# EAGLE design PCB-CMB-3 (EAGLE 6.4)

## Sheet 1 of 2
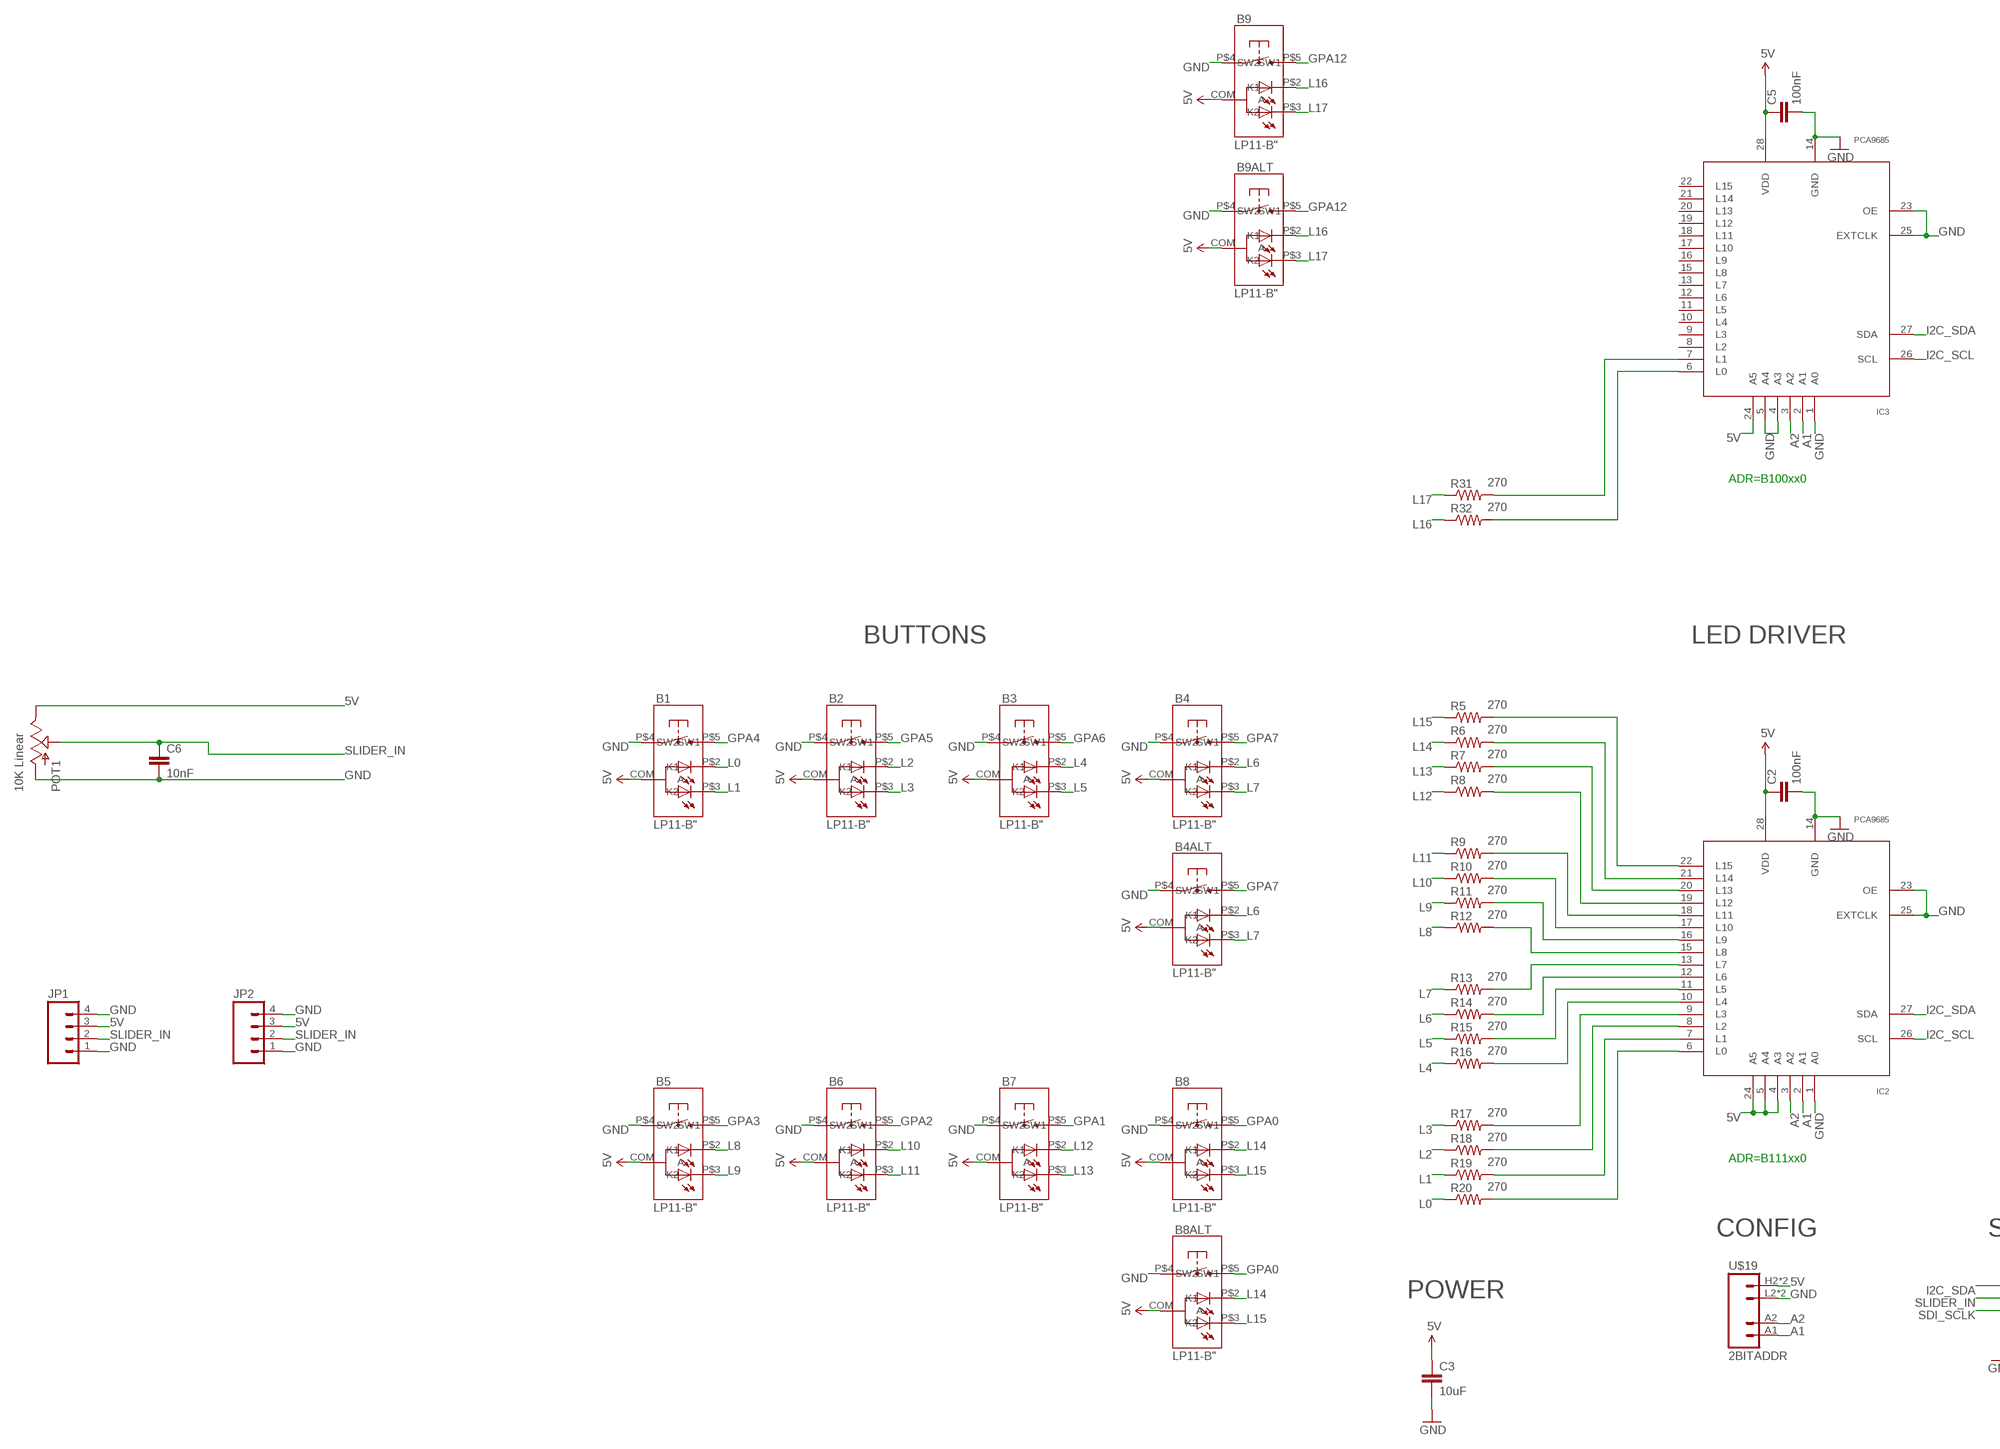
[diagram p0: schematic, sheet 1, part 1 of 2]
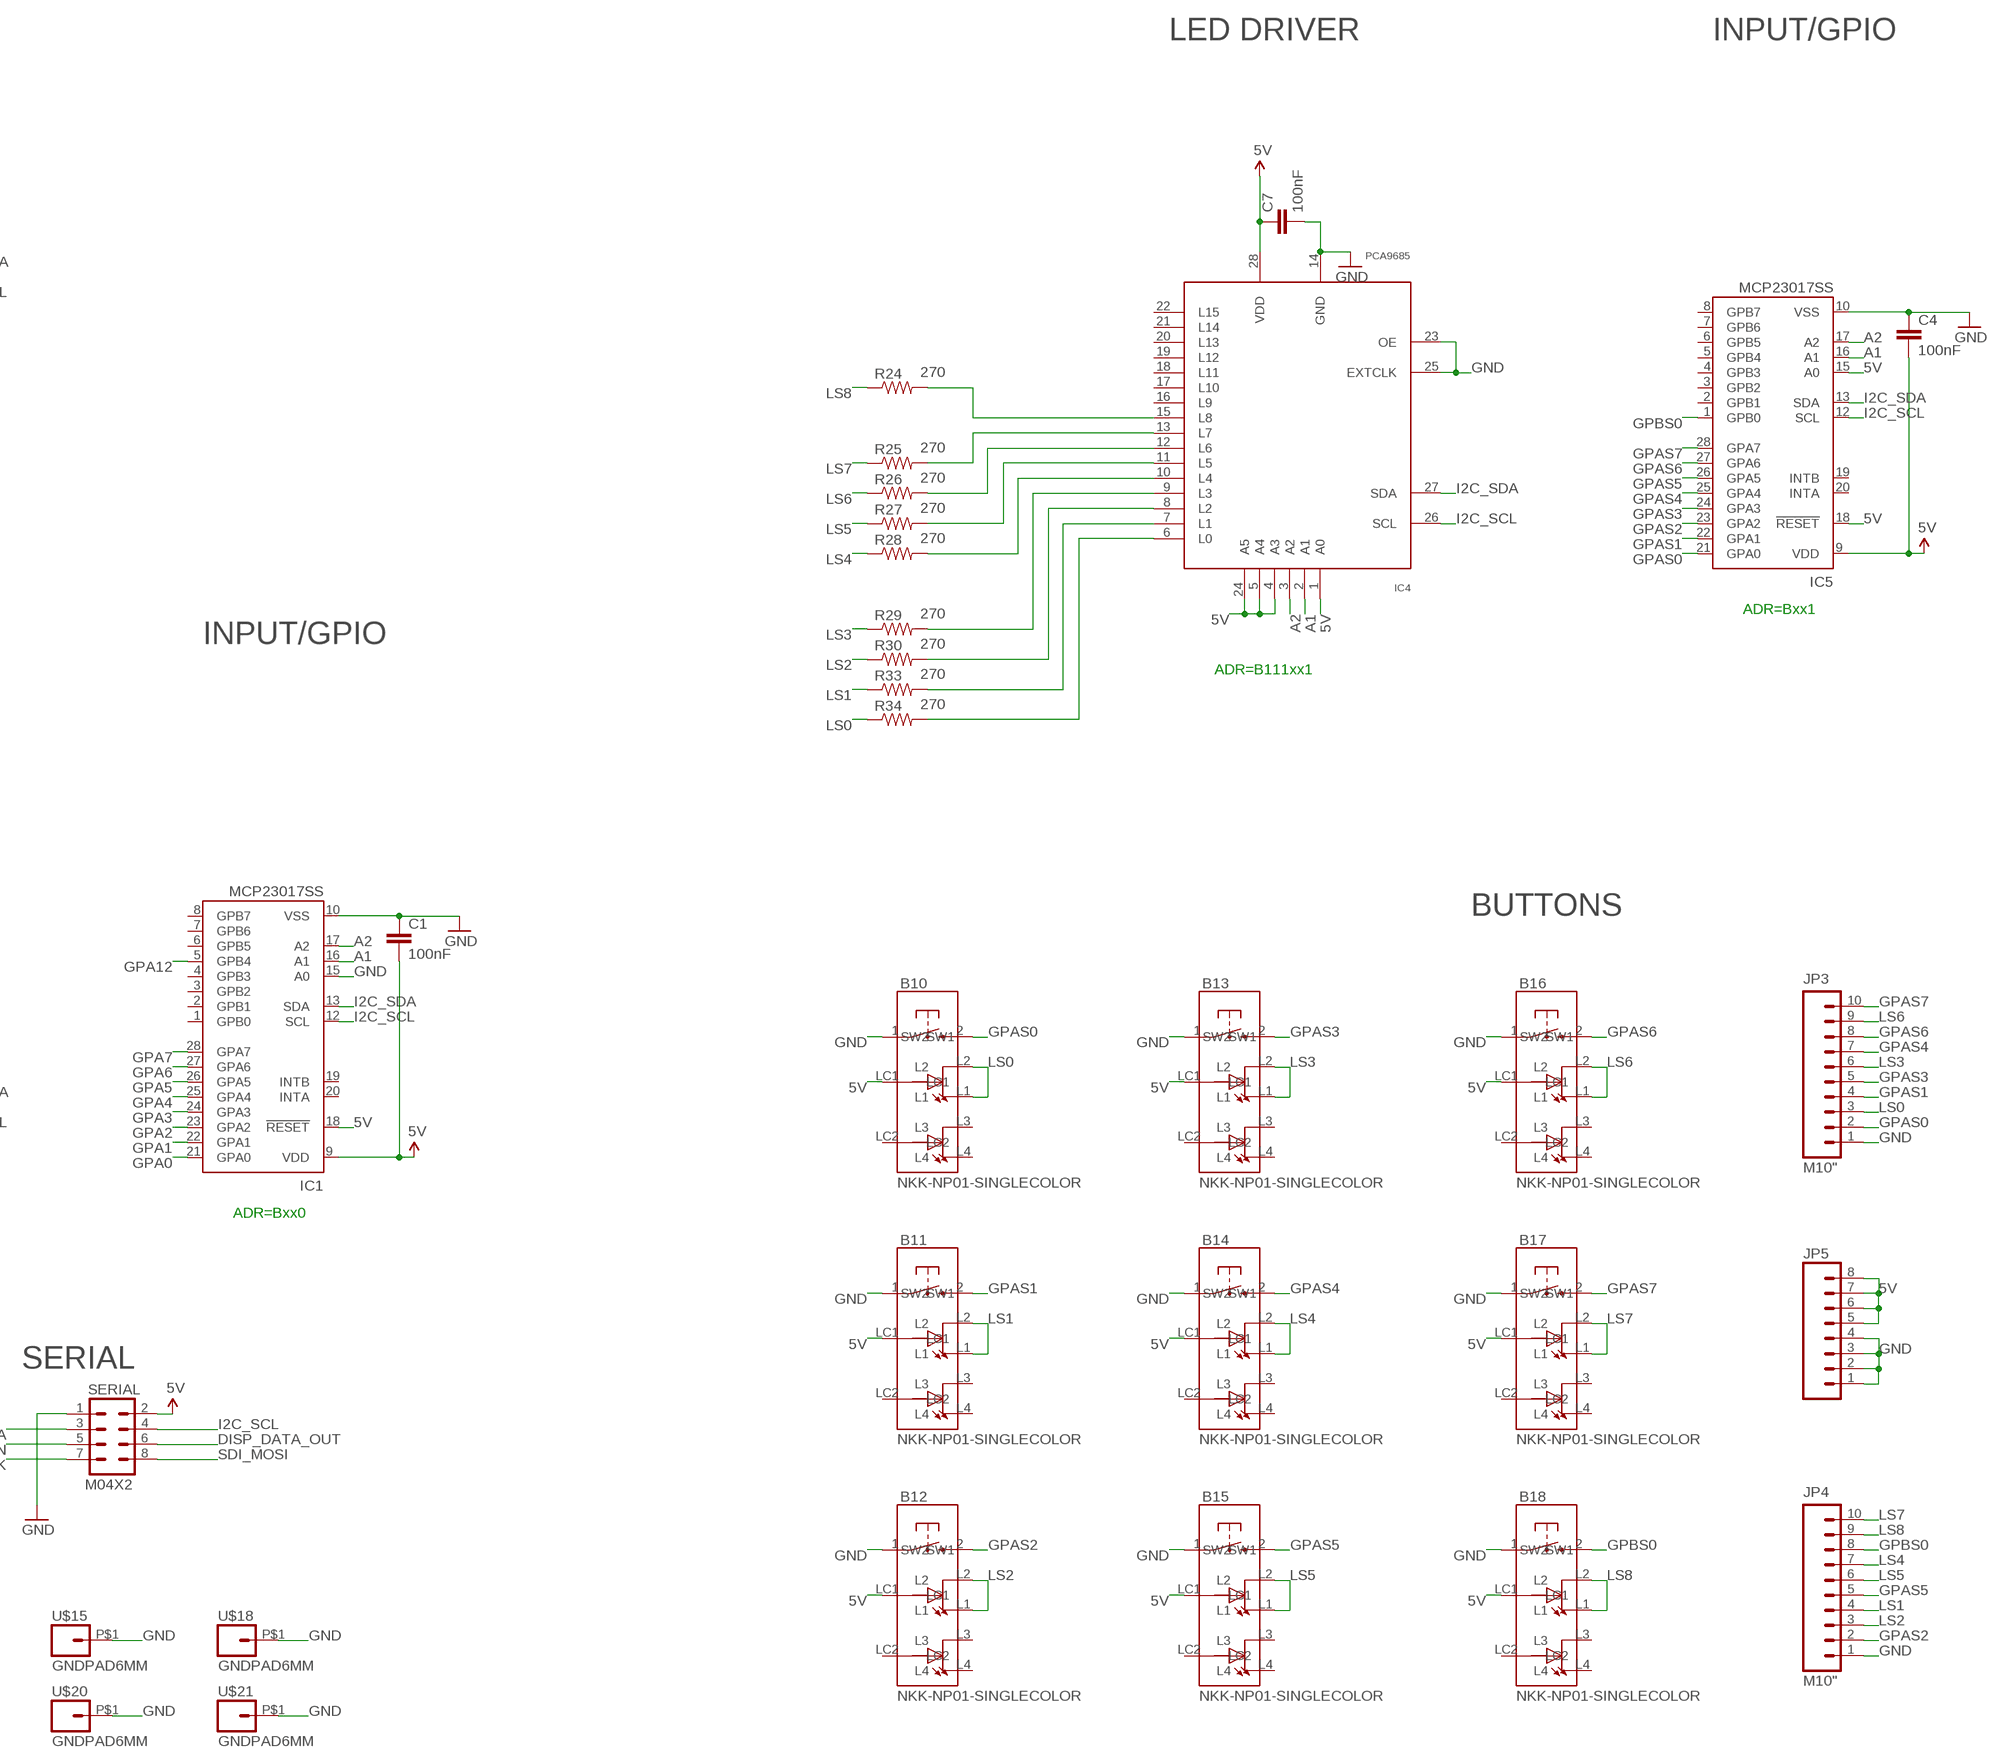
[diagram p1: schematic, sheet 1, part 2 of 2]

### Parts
B1  LP11-B"  [LP11]
B2  LP11-B"  [LP11]
B3  LP11-B"  [LP11]
B4  LP11-B"  [LP11]
B4ALT  LP11-B"  [LP11]
B5  LP11-B"  [LP11]
B6  LP11-B"  [LP11]
B7  LP11-B"  [LP11]
B8  LP11-B"  [LP11]
B8ALT  LP11-B"  [LP11]
B9  LP11-B"  [LP11]
B9ALT  LP11-B"  [LP11]
B10  NKK-NP01-SINGLECOLOR  [NKK-NP01]
B11  NKK-NP01-SINGLECOLOR  [NKK-NP01]
B12  NKK-NP01-SINGLECOLOR  [NKK-NP01]
B13  NKK-NP01-SINGLECOLOR  [NKK-NP01]
B14  NKK-NP01-SINGLECOLOR  [NKK-NP01]
B15  NKK-NP01-SINGLECOLOR  [NKK-NP01]
B16  NKK-NP01-SINGLECOLOR  [NKK-NP01]
B17  NKK-NP01-SINGLECOLOR  [NKK-NP01]
B18  NKK-NP01-SINGLECOLOR  [NKK-NP01]
C1  100nF  CAP0603-CAP  [0603-CAP]
C2  100nF  CAP0603-CAP  [0603-CAP]
C3  10uF  CAP0805  [0805]
C4  100nF  CAP0603-CAP  [0603-CAP]
C5  100nF  CAP0603-CAP  [0603-CAP]
C6  10nF  CAP0603-CAP  [0603-CAP]
C7  100nF  CAP0603-CAP  [0603-CAP]
IC1  MCP23017SS  [SSOP28]
IC2  PCA9685  [TSSOP28]
IC3  PCA9685  [TSSOP28]
IC4  PCA9685  [TSSOP28]
IC5  MCP23017SS  [SSOP28]
JP1  M04PTH  [1X04]
JP2  M04PTH  [1X04]
JP3  M10"  [1X10]
JP4  M10"  [1X10]
JP5  M08LOCK  [1X08_LOCK]
POT1  10K Linear  SLIDER20  [SLIDER20]
R5  270  RESISTOR0603-RES  [0603-RES]
R6  270  RESISTOR0603-RES  [0603-RES]
R7  270  RESISTOR0603-RES  [0603-RES]
R8  270  RESISTOR0603-RES  [0603-RES]
R9  270  RESISTOR0603-RES  [0603-RES]
R10  270  RESISTOR0603-RES  [0603-RES]
R11  270  RESISTOR0603-RES  [0603-RES]
R12  270  RESISTOR0603-RES  [0603-RES]
R13  270  RESISTOR0603-RES  [0603-RES]
R14  270  RESISTOR0603-RES  [0603-RES]
R15  270  RESISTOR0603-RES  [0603-RES]
R16  270  RESISTOR0603-RES  [0603-RES]
R17  270  RESISTOR0603-RES  [0603-RES]
R18  270  RESISTOR0603-RES  [0603-RES]
R19  270  RESISTOR0603-RES  [0603-RES]
R20  270  RESISTOR0603-RES  [0603-RES]
R24  270  RESISTOR0603-RES  [0603-RES]
R25  270  RESISTOR0603-RES  [0603-RES]
R26  270  RESISTOR0603-RES  [0603-RES]
R27  270  RESISTOR0603-RES  [0603-RES]
R28  270  RESISTOR0603-RES  [0603-RES]
R29  270  RESISTOR0603-RES  [0603-RES]
R30  270  RESISTOR0603-RES  [0603-RES]
R31  270  RESISTOR0603-RES  [0603-RES]
R32  270  RESISTOR0603-RES  [0603-RES]
R33  270  RESISTOR0603-RES  [0603-RES]
R34  270  RESISTOR0603-RES  [0603-RES]
SERIAL  M04X2  [2X4]
U$15  GNDPAD6MM  [3.2MMPAD6MM]
U$18  GNDPAD6MM  [3.2MMPAD6MM]
U$19  2BITADDR  [2BITADDR]
U$20  GNDPAD6MM  [3.2MMPAD6MM]
U$21  GNDPAD6MM  [3.2MMPAD6MM]

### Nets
5V [Power]: B1.COM(A) B2.COM(A) B3.COM(A) B4.COM(A) B4ALT.COM(A) B5.COM(A) B6.COM(A) B7.COM(A) B8.COM(A) B8ALT.COM(A) B9.COM(A) B9ALT.COM(A) B10.LC1 B11.LC1 B12.LC1 B13.LC1 B14.LC1 B15.LC1 B16.LC1 B17.LC1 B18.LC1 C1.2 C2.1 C3.1 C4.2 C5.1 C7.1 IC1.9(VDD) IC1.18(!RESET) IC2.4(A3) IC2.5(A4) IC2.24(A5) IC2.28(VDD) IC3.24(A5) IC3.28(VDD) IC4.1(A0) IC4.4(A3) IC4.5(A4) IC4.24(A5) IC4.28(VDD) IC5.9(VDD) IC5.15(A0) IC5.18(!RESET) JP1.3 JP2.3 JP5.5 JP5.6 JP5.7 JP5.8 POT1.1(E) SERIAL.2 U$19.H2(VCC) U$19.H3(VCC)
A1: IC1.16(A1) IC2.2(A1) IC3.2(A1) IC4.2(A1) IC5.16(A1) U$19.A1
A2: IC1.17(A2) IC2.3(A2) IC3.3(A2) IC4.3(A2) IC5.17(A2) U$19.A2
DISP_DATA_OUT: SERIAL.6
GND [Power]: B1.P$4(SW1) B2.P$4(SW1) B3.P$4(SW1) B4.P$4(SW1) B4ALT.P$4(SW1) B5.P$4(SW1) B6.P$4(SW1) B7.P$4(SW1) B8.P$4(SW1) B8ALT.P$4(SW1) B9.P$4(SW1) B9ALT.P$4(SW1) B10.1(SW1) B11.1(SW1) B12.1(SW1) B13.1(SW1) B14.1(SW1) B15.1(SW1) B16.1(SW1) B17.1(SW1) B18.1(SW1) C1.1 C2.2 C3.2 C4.1 C5.2 C6.2 C7.2 IC1.10(VSS) IC1.15(A0) IC2.1(A0) IC2.14(GND) IC2.23(OE) IC2.25(EXTCLK) IC3.1(A0) IC3.4(A3) IC3.5(A4) IC3.14(GND) IC3.23(OE) IC3.25(EXTCLK) IC4.14(GND) IC4.23(OE) IC4.25(EXTCLK) IC5.10(VSS) JP1.1 JP1.4 JP2.1 JP2.4 JP3.1 JP4.1 JP5.1 JP5.2 JP5.3 JP5.4 POT1.3(A) SERIAL.1 U$15.P$1 U$18.P$1 U$19.L2(GND) U$19.L3(GND) U$20.P$1 U$21.P$1
GPA0: B8.P$5(SW2) B8ALT.P$5(SW2) IC1.21(GPA0)
GPA1: B7.P$5(SW2) IC1.22(GPA1)
GPA2: B6.P$5(SW2) IC1.23(GPA2)
GPA3: B5.P$5(SW2) IC1.24(GPA3)
GPA4: B1.P$5(SW2) IC1.25(GPA4)
GPA5: B2.P$5(SW2) IC1.26(GPA5)
GPA6: B3.P$5(SW2) IC1.27(GPA6)
GPA7: B4.P$5(SW2) B4ALT.P$5(SW2) IC1.28(GPA7)
GPA12: B9.P$5(SW2) B9ALT.P$5(SW2) IC1.5(GPB4)
GPAS0: B10.2(SW2) IC5.21(GPA0) JP3.2
GPAS1: B11.2(SW2) IC5.22(GPA1) JP3.4
GPAS2: B12.2(SW2) IC5.23(GPA2) JP4.2
GPAS3: B13.2(SW2) IC5.24(GPA3) JP3.5
GPAS4: B14.2(SW2) IC5.25(GPA4) JP3.7
GPAS5: B15.2(SW2) IC5.26(GPA5) JP4.5
GPAS6: B16.2(SW2) IC5.27(GPA6) JP3.8
GPAS7: B17.2(SW2) IC5.28(GPA7) JP3.10
GPBS0 [Power]: B18.2(SW2) IC5.1(GPB0) JP4.8
I2C_SCL: IC1.12(SCL) IC2.26(SCL) IC3.26(SCL) IC4.26(SCL) IC5.12(SCL) SERIAL.4
I2C_SDA: IC1.13(SDA) IC2.27(SDA) IC3.27(SDA) IC4.27(SDA) IC5.13(SDA) SERIAL.3
L0: B1.P$2(K1) R20.1
L1: B1.P$3(K2) R19.1
L2: B2.P$2(K1) R18.1
L3: B2.P$3(K2) R17.1
L4: B3.P$2(K1) R16.1
L5: B3.P$3(K2) R15.1
L6: B4.P$2(K1) B4ALT.P$2(K1) R14.1
L7: B4.P$3(K2) B4ALT.P$3(K2) R13.1
L8: B5.P$2(K1) R12.1
L9: B5.P$3(K2) R11.1
L10: B6.P$2(K1) R10.1
L11: B6.P$3(K2) R9.1
L12: B7.P$2(K1) R8.1
L13: B7.P$3(K2) R7.1
L14: B8.P$2(K1) B8ALT.P$2(K1) R6.1
L15: B8.P$3(K2) B8ALT.P$3(K2) R5.1
L16: B9.P$2(K1) B9ALT.P$2(K1) R32.1
L17: B9.P$3(K2) B9ALT.P$3(K2) R31.1
LS0: B10.L1 B10.L2 JP3.3 R34.1
LS1: B11.L1 B11.L2 JP4.4 R33.1
LS2: B12.L1 B12.L2 JP4.3 R30.1
LS3: B13.L1 B13.L2 JP3.6 R29.1
LS4: B14.L1 B14.L2 JP4.7 R28.1
LS5: B15.L1 B15.L2 JP4.6 R27.1
LS6: B16.L1 B16.L2 JP3.9 R26.1
LS7: B17.L1 B17.L2 JP4.10 R25.1
LS8: B18.L1 B18.L2 JP4.9 R24.1
N$1: IC4.13(L7) R25.2
N$2: IC4.12(L6) R26.2
N$3: IC4.11(L5) R27.2
N$4: IC2.13(L7) R13.2
N$5: IC2.12(L6) R14.2
N$6: IC4.10(L4) R28.2
N$7: IC2.11(L5) R15.2
N$8: IC4.9(L3) R29.2
N$9: IC2.10(L4) R16.2
N$10: IC2.9(L3) R17.2
N$11: IC2.8(L2) R18.2
N$12: IC2.7(L1) R19.2
N$13: IC4.8(L2) R30.2
N$14: IC3.7(L1) R31.2
N$15: IC3.6(L0) R32.2
N$16: IC4.7(L1) R33.2
N$17: IC4.6(L0) R34.2
N$18: IC4.15(L8) R24.2
N$19: IC2.6(L0) R20.2
N$20: IC2.15(L8) R12.2
N$21: IC2.16(L9) R11.2
N$22: IC2.17(L10) R10.2
N$23: IC2.18(L11) R9.2
N$24: IC2.19(L12) R8.2
N$25: IC2.20(L13) R7.2
N$26: IC2.21(L14) R6.2
N$27: IC2.22(L15) R5.2
SDI_MOSI: SERIAL.8
SDI_SCLK: SERIAL.7
SLIDER_IN: C6.1 JP1.2 JP2.2 POT1.2A(S) SERIAL.5
Unconnected: B10.L3 B10.L4 B10.LC2 B11.L3 B11.L4 B11.LC2 B12.L3 B12.L4 B12.LC2 B13.L3 B13.L4 B13.LC2 B14.L3 B14.L4 B14.LC2 B15.L3 B15.L4 B15.LC2 B16.L3 B16.L4 B16.LC2 B17.L3 B17.L4 B17.LC2 B18.L3 B18.L4 B18.LC2 IC1.1(GPB0) IC1.2(GPB1) IC1.3(GPB2) IC1.4(GPB3) IC1.6(GPB5) IC1.7(GPB6) IC1.8(GPB7) IC1.19(INTB) IC1.20(INTA) IC3.8(L2) IC3.9(L3) IC3.10(L4) IC3.11(L5) IC3.12(L6) IC3.13(L7) IC3.15(L8) IC3.16(L9) IC3.17(L10) IC3.18(L11) IC3.19(L12) IC3.20(L13) IC3.21(L14) IC3.22(L15) IC4.16(L9) IC4.17(L10) IC4.18(L11) IC4.19(L12) IC4.20(L13) IC4.21(L14) IC4.22(L15) IC5.2(GPB1) IC5.3(GPB2) IC5.4(GPB3) IC5.5(GPB4) IC5.6(GPB5) IC5.7(GPB6) IC5.8(GPB7) IC5.19(INTB) IC5.20(INTA)

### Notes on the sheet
- LED DRIVER | INPUT/GPIO
- ADR=B100xx0
- ADR=Bxx1
- BUTTONS | LED DRIVER | INPUT/GPIO
- ADR=B111xx1
- BUTTONS
- ADR=Bxx0
- ADR=B111xx0
- CONFIG | SERIAL
- POWER

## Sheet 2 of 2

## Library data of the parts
B1-B4 B4ALT B5-B8 B8ALT B9 B9ALT = SKAARHOJ:LP11-B
B10-B18 = SKAARHOJ:NKK-NP01-SINGLECOLOR
C1-C7 = SparkFun:CAP: Capacitor
IC1 IC5 = microchip:MCP23017: http://ww1.microchip.com/downloads/en/DeviceDoc/21952a.pdf Source: http://ww1.microchip.com/downloads/en/DeviceDoc/21952a.pdf; MF: MICROCHIP; MPN: MCP23017-E/SS; OC_FARNELL: 1467674; OC_NEWARK: 31K2960
IC2-IC4 = wsmith:PCA9685
JP1 JP2 = SparkFun:M04: Header 4 Standard 4-pin 0.1" header. Use with straight break away headers (SKU : PRT-00116), right angle break away headers (PRT-00553), swiss pins (PRT-00743), machine pins (PRT-00117), and female headers (PRT-00115). Molex polarized connector foot print use with SKU : PRT-08231 with associated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
JP3 JP4 = SparkFun:M10: Header 10 Standard 10-pin 0.1" header. Use with straight break away headers (SKU : PRT-00116), right angle break away headers (PRT-00553), swiss pins (PRT-00743), machine pins (PRT-00117), and female headers (PRT-00115).
JP5 = SparkFun:M08: Header 8 Standard 8-pin 0.1" header. Use with straight break away headers (SKU : PRT-00116), right angle break away headers (PRT-00553), swiss pins (PRT-00743), machine pins (PRT-00117), and female headers (PRT-00115).
POT1 = SKAARHOJ:SLIDER
R5-R20 R24-R34 = SparkFun:RESISTOR: Resistor
SERIAL = SparkFun:M04X2
U$15 U$18 U$20 U$21 = SKAARHOJ:GNDPAD
U$19 = SKAARHOJ:2BITADDR

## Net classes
0 default: width 0.203 mm, drill 0.406 mm, clearance 0.203 mm
1 Power: width 0.406 mm, drill 0.61 mm, clearance 0.203 mm

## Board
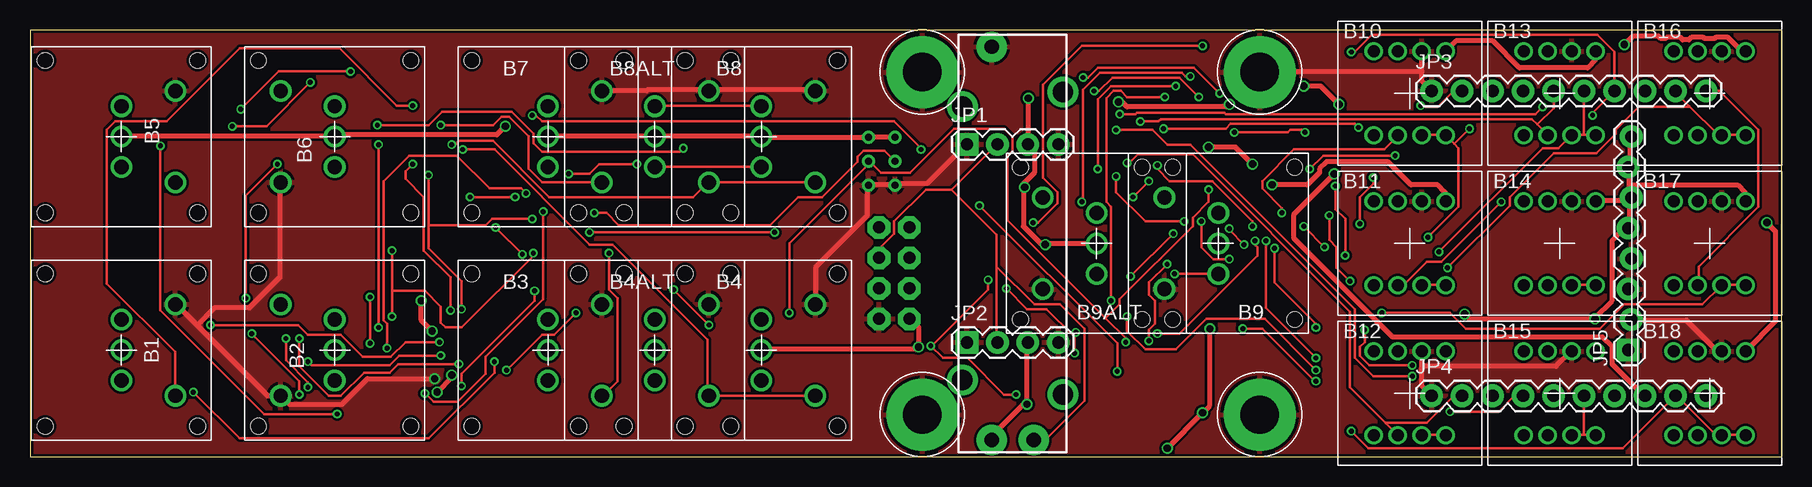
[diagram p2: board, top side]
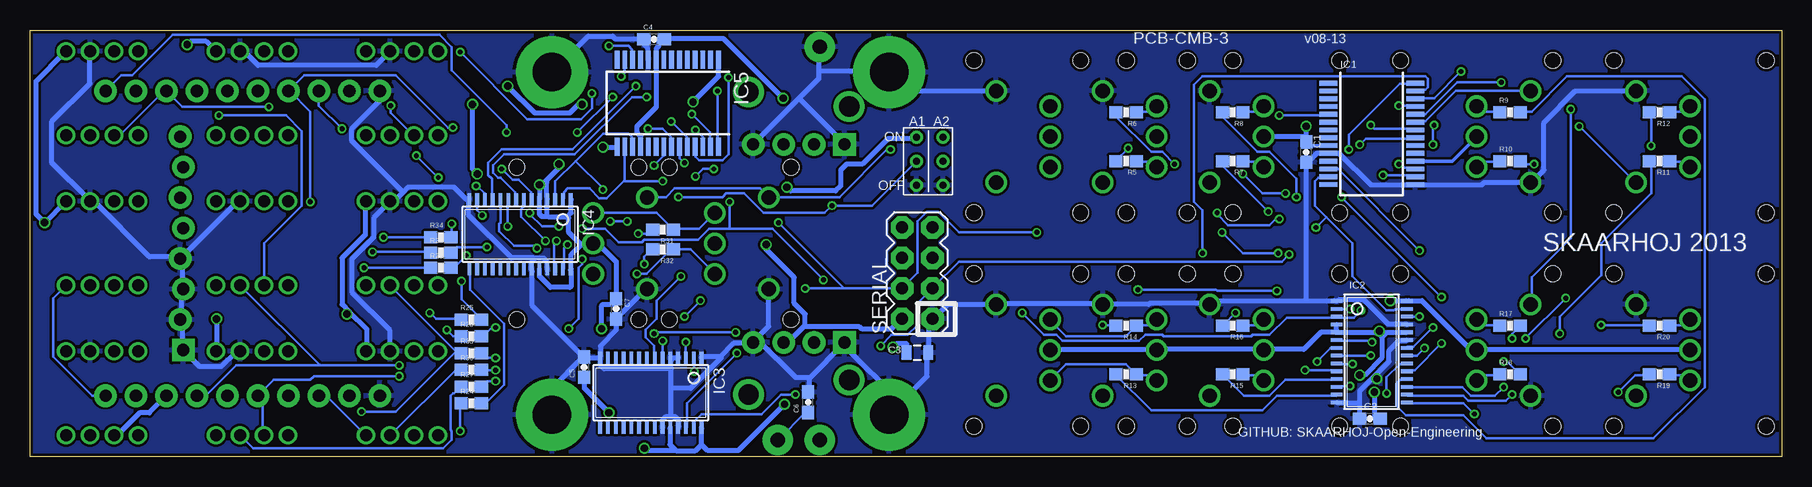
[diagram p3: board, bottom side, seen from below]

Size 146 x 35.56 mm. Coordinates in mm from the lower left corner, seen from the top.
Outline: 0,0 146,0 146,35.56 0,35.56 0,0
Copper layers (1*16): Top 0.035mm / dielectric 1.5mm / Bottom 0.035mm
Design rules "Fusion_eagle_rule_v1.1": minimum track width 6mil, minimum drill 12mil, track to track 6mil, track to pad 6mil, pad to pad 6mil, via to via 6mil, smd to smd 0mil, copper to edge 10mil, drill to drill 10mil, minimum pad ring 10mil, minimum via ring 6mil, stop-mask expansion 2mil, vias tented up to drill 100mil, thermal gap 10mil

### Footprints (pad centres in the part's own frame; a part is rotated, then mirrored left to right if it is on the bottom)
LP11 = drill 1.2: COM 0,0; P$2 0,2.54; P$3 0,-2.54; P$4 4.5,3.81; P$5 4.5,-3.81 | hole 1.3: -6.35,6.35; 6.35,6.35; 6.35,-6.35; -6.35,-6.35
NKK-NP01 = drill 1: 1 1,3.5; 2 -1,-3.5; L1 3,-3.5; L2 1,-3.5; L3 -1,3.5; L4 -3,3.5; LC1 3,3.5; LC2 -3,-3.5
0603-CAP = smd 1.1 x 1: 1 -0.85,0; 2 0.85,0
0805 = smd 0.8 x 1.2: 1 -0.9,0; 2 0.9,0
SSOP28 = smd 0.4 x 1.5: 1 -4.225,-3.625; 2 -3.575,-3.625; 3 -2.925,-3.625; 4 -2.275,-3.625; 5 -1.625,-3.625; 6 -0.975,-3.625; 7 -0.325,-3.625; 8 0.325,-3.625; 9 0.975,-3.625; 10 1.625,-3.625; 11 2.275,-3.625; 12 2.925,-3.625; 13 3.575,-3.625; 14 4.225,-3.625; 15 4.225,3.625; 16 3.575,3.625; 17 2.925,3.625; 18 2.275,3.625; 19 1.625,3.625; 20 0.975,3.625; 21 0.325,3.625; 22 -0.325,3.625; 23 -0.975,3.625; 24 -1.625,3.625; 25 -2.275,3.625; 26 -2.925,3.625; 27 -3.575,3.625; 28 -4.225,3.625
TSSOP28 = smd 0.305 x 0.991: 1 -4.225,-2.918; 2 -3.575,-2.918; 3 -2.925,-2.918; 4 -2.275,-2.918; 5 -1.625,-2.918; 6 -0.975,-2.918; 7 -0.325,-2.918; 8 0.325,-2.918; 9 0.975,-2.918; 10 1.625,-2.918; 11 2.275,-2.918; 12 2.925,-2.918; 13 3.575,-2.918; 14 4.225,-2.918; 15 4.225,2.918; 16 3.575,2.918; 17 2.925,2.918; 18 2.275,2.918; 19 1.625,2.918; 20 0.975,2.918; 21 0.325,2.918; 22 -0.325,2.918; 23 -0.975,2.918; 24 -1.625,2.918; 25 -2.275,2.918; 26 -2.925,2.918; 27 -3.575,2.918; 28 -4.225,2.918
1X04 = drill 1.016 pad 1.88 square: 1 0,0 | drill 1.016 pad 1.88: 2 2.54,0; 3 5.08,0; 4 7.62,0
1X10 = drill 1.016 pad 1.88: 1 0,0; 2 2.54,0; 3 5.08,0; 4 7.62,0; 5 10.16,0; 6 12.7,0; 7 15.24,0; 8 17.78,0; 9 20.32,0; 10 22.86,0
1X08_LOCK = drill 1.016 pad 1.88 square: 1 0,0.127 | drill 1.016 pad 1.88: 2 2.54,-0.127; 3 5.08,0.127; 4 7.62,-0.127; 5 10.16,0.127; 6 12.7,-0.127; 7 15.24,0.127; 8 17.78,-0.127
SLIDER20 = drill 1.194 pad 2.54: 1 -16.383,1.74; 2A -16.383,-1.74; 3 16.383,1.74 | drill 1.702: P$1 -11.392,4.191; P$2 11.392,4.191; P$3 12.598,-4.191; P$4 -12.598,-4.191
0603-RES = smd 1.1 x 1: 1 -0.85,0; 2 0.85,0
2X4 = drill 1.016 pad 1.88 octagon: 1 -3.81,-1.27; 2 -3.81,1.27; 3 -1.27,-1.27; 4 -1.27,1.27; 5 1.27,-1.27; 6 1.27,1.27; 7 3.81,-1.27; 8 3.81,1.27
3.2MMPAD6MM = drill 3.2 pad 6: P$1 0,0
2BITADDR = drill 0.6: A1 0,0; A2 2.2,0; H2 0,2; H3 2.2,2; L2 0,-2; L3 2.2,-2

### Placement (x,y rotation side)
B1  7.62,8.89 0 top
B2  25.4,8.89 180 top
B3  43.18,8.89 0 top
B4  60.96,8.89 0 top
B4ALT  52.07,8.89 0 top
B5  7.62,26.67 0 top
B6  25.4,26.67 180 top
B7  43.18,26.67 0 top
B8  60.96,26.67 0 top
B8ALT  52.07,26.67 0 top
B9  99.06,17.78 180 top
B9ALT  88.9,17.78 180 top
B10  115,30.28 0 top
B11  115,17.78 0 top
B12  115,5.28 0 top
B13  127.5,30.28 0 top
B14  127.5,17.78 0 top
B15  127.5,5.28 0 top
B16  140,30.28 0 top
B17  140,17.78 0 top
B18  140,5.28 0 top
C1  39.62,25.38 90 bottom
C2  34.32,3.16 180 bottom
C3  72.04,8.67 0 bottom
C4  93.98,34.8 0 bottom
C5  99.81,7.47 90 bottom
C6  81.13,4.54 90 bottom
C7  97.16,12.32 270 bottom
IC1  34.16,26.91 270 bottom
IC2  34.16,8.75 270 bottom
IC3  94.25,5.33 180 bottom
IC4  105.16,18.54 180 bottom
IC5  92.84,29.46 180 bottom
JP1  78.11,26.04 0 top
JP2  78.11,9.53 0 top
JP3  116.84,30.48 0 top
JP4  116.84,5.08 0 top
JP5  133.35,8.89 90 top
POT1  81.92,17.78 90 top
R5  54.63,24.64 180 bottom
R6  54.63,28.7 180 bottom
R7  45.74,24.64 180 bottom
R8  45.74,28.7 180 bottom
R9  22.62,28.7 0 bottom
R10  22.62,24.64 0 bottom
R11  10.18,24.64 180 bottom
R12  10.18,28.7 180 bottom
R13  54.63,6.86 180 bottom
R14  54.63,10.92 180 bottom
R15  45.74,6.86 180 bottom
R16  45.74,10.92 180 bottom
R17  22.62,10.92 0 bottom
R18  22.62,6.86 0 bottom
R19  10.18,6.86 180 bottom
R20  10.18,10.92 180 bottom
R24  109.22,4.45 0 bottom
R25  109.22,11.43 0 bottom
R26  111.76,15.75 0 bottom
R27  109.22,5.84 0 bottom
R28  109.22,10.03 0 bottom
R29  111.76,17.02 0 bottom
R30  109.22,7.24 0 bottom
R31  93.23,18.92 180 bottom
R32  93.23,17.27 180 bottom
R33  109.22,8.64 0 bottom
R34  111.76,18.29 0 bottom
SERIAL  72.04,15.3 90 bottom
U$15  74.39,3.5 0 top
U$18  102.5,3.5 0 top
U$19  72.1,24.62 0 bottom
U$20  74.39,32.06 0 top
U$21  102.5,32.06 0 top

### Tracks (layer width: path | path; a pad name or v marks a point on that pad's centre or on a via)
5V  (via drill 0.61)
  Top 0.406: B10.LC1 118.06,33.83 118.87,34.65 121.92,34.65 124.16,32.41 129.84,32.41 130.45,33.02 130.45,33.73 B13.LC1 | v144.78,19.51 145.49,18.8 145.49,11.28 143.05,8.84 B18.LC1 | v132.89,34.34 133.6,35.05 135.74,35.05 135.94,34.85 136.35,34.85 136.45,34.95 137.57,34.95 137.77,34.75 138.28,34.75 138.48,34.95 139.5,34.95 139.6,34.85 140.41,34.85 140.51,34.95 141.53,34.95 142.65,33.83 142.95,33.83 B16.LC1 | v98.25,25.81 100.48,25.81 v101.91,24.38 | B14.LC1 130.56,21.34 133.2,21.34 133.4,21.54 JP5.6 | JP5.6 133.3,21.23 133.3,19.1 JP5.5 133.1,18.9 132.79,18.9 131.88,17.98 131.88,13.01 130.45,11.58 v130.45,11.48 119.99,11.48 v119.58,11.89 | 133.3,22.66 133.3,21.64 JP5.6 | 133.3,22.66 133.3,24.08 JP5.7 133.4,24.18 133.4,26.62 JP5.8 | v103.53,22.66 106.48,22.66 107.49,23.67 107.49,23.98 108.1,24.59 113.18,24.59 115.11,22.66 117.35,22.66 117.96,22.05 117.96,21.34 B11.LC1 | 133.3,22.66 142.34,22.66 142.95,22.05 142.95,21.34 B17.LC1 | v32.61,13.01 32.61,11.38 v33.53,10.46 | v33.93,5.38 35.15,6.6 v35.15,6.81 | 84.63,17.78 84.23,17.78 82.8,19.2 82.8,22.45 | 84.63,17.78 B9ALT.COM | 82.8,22.45 82.8,22.76 83.72,23.67 83.72,25.5 JP1.3 83.21,26.21 v83.21,29.87 | v94.79,0.71 v97.74,3.66 98.35,4.27 v98.35,10.67 | SERIAL.2 73.36,11.48 74.07,10.77 v74.07,9.14 73.86,8.94 60.96,8.94 B4.COM | 82.91,4.47 80.26,1.83 80.26,1.42 POT1.1 | 82.91,4.47 83.11,4.67 83.11,9.45 JP2.3 | v83.11,4.37 83.01,4.37 82.91,4.47 | v84.63,17.68 84.63,17.78 | B5.COM 7.62,26.72 25.4,26.72 B6.COM 25.5,26.82 38.91,26.82 v39.62,27.53 | U$19.H2 72.03,26.62 70,26.62 U$19.H3 69.8,26.62 60.96,26.62 B8.COM 60.86,26.72 52.12,26.72 B8ALT.COM 51.92,26.72 43.18,26.72 B7.COM
  Top 0.406: v82.91,22.45 82.8,22.45
  Bottom 0.305: IC1.9 39.62,25.93 C1.2 | IC1.18 27.44,24.63 B6.COM
  Bottom 0.406: B17.LC1 143.05,21.23 v144.78,19.51 145.49,20.22 145.49,31.29 143.05,33.73 B16.LC1 | v132.89,34.34 132.59,34.65 131.37,34.65 130.56,33.83 B13.LC1 | 101.19,20.02 100.89,20.32 100.89,21.44 IC4.1 | 101.19,20.02 102.82,20.02 102.92,20.12 | 102.92,20.12 102.92,21.44 IC4.4 102.92,21.64 102.92,22.86 103.02,22.96 101.91,24.08 v101.91,24.38 | 102.92,20.12 103.02,20.02 103.33,20.02 103.53,20.22 103.53,21.44 IC4.5 103.53,21.64 v103.53,22.66 | v98.25,25.81 97.13,25.81 IC5.15 | 100.08,17.68 100.89,16.87 100.89,15.65 IC4.28 100.89,15.44 100.89,14.22 100.99,14.12 102.62,14.12 103.53,15.04 103.53,15.54 IC4.24 | 100.08,17.68 99.97,17.78 B9.COM 98.96,17.68 98.55,17.68 97.13,16.26 97.13,13.21 C7.1 97.13,13.01 97.13,12.7 98.25,12.7 98.35,12.6 v98.35,10.67 | 100.08,17.68 101.09,18.69 101.09,19.91 101.19,20.02 | 119.38,12.09 119.99,12.7 119.99,16.56 118.06,18.49 118.06,21.23 B11.LC1 | 119.38,12.09 117.96,10.67 117.96,8.84 B12.LC1 | v130.45,11.48 130.45,8.84 B15.LC1 | v119.58,11.89 119.38,12.09 | B1.COM 7.62,8.94 25.4,8.94 B2.COM 25.5,9.04 26.01,9.04 29.97,13.01 31.09,13.01 IC2.28 31.29,13.01 v32.61,13.01 | B4.COM 60.96,8.94 52.12,8.94 B4ALT.COM 51.92,8.94 43.28,8.94 B3.COM 43.18,8.94 39.83,8.94 38.41,10.36 37.19,10.36 IC2.5 | 33.53,10.36 36.98,10.36 IC2.5 | 33.53,10.36 33.02,10.36 | 33.02,10.36 31.29,10.36 IC2.24 | v33.53,10.46 33.53,10.36 | IC2.4 37.08,10.97 37.08,10.57 IC2.5 | v33.93,5.38 33.93,3.15 33.53,3.15 C2.1 | v35.15,6.81 34.75,6.81 33.33,8.23 33.33,9.96 33.02,10.26 33.02,10.36 | IC5.18 95.1,25.91 95.1,26.72 95.4,27.03 95.4,27.53 93.78,29.16 93.78,32.92 IC5.9 93.78,33.12 93.78,34.04 93.57,34.24 93.57,34.85 93.17,34.85 C4.2 92.96,34.85 88.19,34.85 v83.21,29.87
  Bottom 0.406: 90.02,1.02 90.02,2.34 IC3.28 | 90.02,1.02 90.53,0.51 92.15,0.51 92.25,0.61 | 92.25,0.61 92.66,1.02 92.66,2.34 IC3.24 | v97.74,3.66 99.77,5.69 99.77,6.6 C5.1 | v94.79,0.71 94.59,0.51 92.35,0.51 92.25,0.61 | v74.07,9.14 73.76,9.45 72.95,9.45 72.95,8.74 C3.1 | 81.38,10.87 81.48,10.87 82.8,9.55 83.11,9.55 JP2.3 | 81.38,10.87 76.91,10.87 76.71,10.67 74.17,10.67 73.36,11.48 SERIAL.2 | 90.02,1.02 89.51,0.51 86.97,0.51 v83.11,4.37 | v84.63,17.68 84.63,17.27 82.3,14.94 82.3,12.8 81.38,11.89 81.38,10.87 | 39.62,26.72 C1.2 | 39.62,26.72 43.18,26.72 B7.COM | 39.62,26.72 v39.62,27.53 | v82.91,22.45 82.6,22.15 78.84,22.15 78.44,22.55 78.44,23.88 77.93,24.38 76.61,24.38 74.47,26.52 72.14,26.52 U$19.H2
A1  (via drill 0.41)
  Top 0.203: v35.97,12.29 35.97,14.63 33.22,17.37 33.22,19.3 | v33.22,23.47 33.22,19.3 | v90.63,7.11 90.63,9.45 v79.15,20.93 | v91.95,21.64 v93.27,22.96 | 33.22,19.3 38,19.3 38.51,19.81 v41.86,19.81 | v47.04,20.32 48.06,20.32 49.07,19.3 61.67,19.3 64.01,21.64 66.04,21.64 68.99,24.59 68.99,24.99 69.49,25.5 71.22,25.5 72.03,24.69 U$19.A1
  Bottom 0.203: v35.97,12.29 36.98,12.29 IC2.2 | v33.22,23.47 30.68,23.47 30.58,23.37 IC1.16 | 96.47,23.01 96.42,23.06 96.42,25.81 IC5.16 | 96.47,23.01 97.94,21.54 98.55,21.54 99.36,22.35 101.19,22.35 101.5,22.05 101.5,21.54 IC4.2 | v90.63,7.11 90.63,8.23 IC3.2 | U$19.A1 72.14,24.59 75.79,20.93 v79.15,20.93 79.76,20.32 84.84,20.32 86.46,21.95 87.99,21.95 88.29,21.64 v91.95,21.64 | v93.27,22.96 96.42,22.96 96.47,23.01 | v41.86,19.81 42.16,19.81 42.67,19.3 46.13,19.3 47.04,20.22 v47.04,20.32
A2  (via drill 0.41)
  Top 0.203: v35.05,12.19 35.05,14.94 32.82,17.17 32.82,21.64 31.29,23.16 31.29,23.77 v31.9,24.38 | v91.34,9.55 91.34,9.86 89.66,11.53 | 89.66,11.53 81.48,19.71 81.48,25.09 81.89,25.5 81.89,26.62 81.18,27.33 77.01,27.33 73.36,23.67 70.92,23.67 70,24.59 U$19.A2 70,24.49 63.3,17.78 v63.3,11.99 | v98.25,22.25 98.25,21.23 96.93,19.91 96.93,19.2 90.83,13.11 90.83,12.7 89.66,11.53
  Bottom 0.203: v35.05,12.19 35.66,11.58 36.98,11.58 IC2.3 37.08,11.58 41.25,11.58 42.67,10.16 44.09,10.16 44.2,10.06 51.51,10.06 51.61,10.16 53.03,10.16 53.54,9.65 59.94,9.65 60.45,10.16 61.47,10.16 v63.3,11.99 | v31.9,24.38 31.7,24.38 31.39,24.08 30.58,24.08 IC1.17 | 100.53,24.64 98.25,26.92 96.11,26.92 95.81,26.62 95.81,25.91 IC5.17 | 100.53,24.64 102.21,22.96 102.21,21.54 IC4.3 | v91.34,9.55 91.34,8.33 IC3.3 | 100.53,24.64 98.25,22.35 v98.25,22.25
GND  (via drill 0.61)
  Top 0.406: 116.03,7.52 116.03,5.89 JP4.1 | 116.03,7.52 116.03,8.74 B12.1 | 116.03,7.52 127.2,7.52 128.42,8.74 B15.1 | B18.1 140.92,8.84 140.61,8.84 138.07,11.38 133.5,11.38 JP5.2 | 116.03,32.11 116.03,31.29 JP3.1 | 116.03,32.11 116.03,33.73 B10.1 | 116.03,32.11 102.51,32.11 U$21.P$1 | JP1.1 78.03,26.01 74.78,22.76 72.24,22.76 U$19.L2 72.03,22.66 70,22.66 U$19.L3 69.8,22.45 69.8,20.12 65.53,15.85 65.53,12.7 B4.P$4 | B7.P$4 51.41,30.48 51.51,30.58 56.39,30.58 56.49,30.48 B8ALT.P$4 56.69,30.58 65.33,30.58 65.43,30.48 B8.P$4 | 13.92,10.97 12.19,12.7 B1.P$4 | 13.92,10.97 19.81,5.08 B2.P$4 21.03,4.98 21.64,4.37 26.01,4.37 28.14,6.5 v33.73,6.5 | 13.92,10.97 15.34,12.39 18.29,12.39 20.83,14.94 20.83,22.86 B6.P$4
  Bottom 0.406: B15.1 128.52,8.74 128.83,8.74 130.05,7.52 131.88,7.52 133.2,8.84 JP5.1 133.3,9.04 133.3,11.38 JP5.2 133.4,11.48 133.4,13.92 JP5.3 133.3,14.02 133.3,16.46 JP5.4 | B14.1 128.52,21.23 128.73,21.23 133.4,16.56 JP5.4 | JP5.4 133.6,16.66 136.04,16.66 140.61,21.23 140.92,21.23 B17.1 141.12,21.44 144.17,24.49 144.17,27.94 141.02,31.09 141.02,33.73 B16.1 | B13.1 128.42,33.73 128.12,33.73 127,32.61 117.14,32.61 116.03,33.73 B10.1 | IC5.10 94.49,33.12 94.49,34.04 94.79,34.34 94.79,34.75 C4.1 95,34.85 97.23,34.85 97.43,35.05 99.47,35.05 102.41,32.11 U$21.P$1 | 103.94,16.46 104.24,16.15 104.24,15.65 IC4.23 104.14,15.44 104.14,12.6 99.97,8.43 C5.2 | 103.94,16.46 103.83,16.56 103.23,16.56 102.92,16.26 102.92,15.65 IC4.25 | 103.94,16.46 104.04,16.56 105.87,16.56 109.42,20.12 109.42,21.23 IC4.14 109.42,21.44 109.63,21.44 110.64,22.45 114.5,22.45 114.91,22.05 | 114.91,22.05 115.62,21.34 115.93,21.34 B11.1 116.13,21.13 117.35,19.91 117.35,18.29 119.18,16.46 119.18,13.72 116.03,10.57 116.03,8.84 B12.1 | 98.45,8.23 IC3.14 | IC3.14 98.65,8.23 99.77,8.23 C5.2 | B9.P$4 94.59,14.02 97.13,11.48 C7.2 97.13,11.28 97.13,10.57 98.45,9.25 98.45,8.43 IC3.14 | C5.2 99.97,8.23 102.41,5.79 102.41,3.56 U$18.P$1 | JP3.1 116.84,29.67 119.18,27.33 119.18,26.31 114.91,22.05 | 81.89,29.87 80.26,31.5 80.26,32.11 | 81.89,29.87 JP1.4 | 80.26,32.11 80.26,34.14 POT1.3 | 81.89,29.87 78.13,26.11 JP1.1 | B8.P$4 72.85,30.48 74.37,32 U$20.P$1 74.57,32.11 80.26,32.11 | 33.93,6.71 35.15,5.49 35.15,4.47 | 33.93,6.71 32.72,7.92 32.72,8.84 31.9,9.65 31.29,9.65 IC2.23 | 35.15,4.47 35.15,3.25 C2.2
  Bottom 0.406: 35.15,4.47 36.98,4.47 IC2.14 | v33.73,6.5 33.93,6.71 | B5.P$4 17.17,30.48 19.81,27.84 19.81,23.88 20.73,22.96 B6.P$4 24.79,22.86 24.99,22.66 30.38,22.66 IC1.15 30.58,22.66 34.24,22.66 36.88,25.3 37.59,25.3 IC1.10 37.8,25.3 38.71,25.3 39.42,24.59 39.62,24.59 C1.1 39.62,13.01 | IC2.25 31.29,11.07 32.82,11.07 34.85,13.11 36.88,13.11 36.98,13.01 IC2.1 37.29,13.01 39.62,13.01 | 39.62,13.01 47.35,13.01 47.65,12.7 B3.P$4 47.85,12.8 52.63,12.8 52.73,12.7 B4ALT.P$4 56.69,12.8 65.33,12.8 B4.P$4 69.49,12.7 70.61,11.58 SERIAL.1 70.81,11.48 71.12,11.18 71.12,8.74 C3.2 71.22,8.53 71.22,6.71 74.37,3.56 U$15.P$1 73.46,4.57 78.13,9.25 JP2.1 78.13,9.45 81.08,6.5 | 81.08,6.5 81.08,5.49 C6.2 | IC3.4 92.05,8.23 92.56,8.23 IC3.5 92.56,8.03 92.56,7.32 | 92.56,3.35 92.96,3.35 93.27,3.05 93.27,2.44 IC3.23 | 92.56,3.35 92.25,3.35 91.95,3.05 91.95,2.44 IC3.25 | 92.56,3.35 92.56,5.69 | 92.56,5.69 92.56,7.32 | 88.49,8.33 90.02,8.33 IC3.1 | 88.49,8.33 87.38,9.45 85.75,9.45 JP2.4 | 92.56,5.69 90.93,5.69 88.39,8.23 88.49,8.33 | B9ALT.P$4 84.43,13.92 84.43,10.87 85.65,9.65 JP2.4 | 81.08,6.5 81.18,6.6 82.19,6.6 85.34,9.75 JP2.4 | 92.56,7.32 98.15,7.32 98.45,7.62 98.45,8.03 IC3.14
  pour Top: 0,0 146.05,0 146.05,35.56 0,35.56
  pour Bottom: 0,0 146.05,0 146.05,35.56 0,35.56
GPA0  (via drill 0.41)
  Top 0.203: v35.15,26.01 35.46,26.01 35.76,26.31 38.61,26.31 43.28,21.64 55.27,21.64 56.49,22.86 B8ALT.P$5 B8.P$5
  Bottom 0.203: v35.15,26.01 34.65,26.52 30.58,26.52 IC1.21
GPA1  (via drill 0.41)
  Top 0.203: v34.24,27.64 38.61,27.64 39.32,28.35 39.93,28.35 41.55,26.72 41.55,23.98 42.67,22.86 B7.P$5
  Bottom 0.203: v34.24,27.64 33.93,27.33 30.58,27.33 IC1.22
GPA2
  Bottom 0.203: B6.P$5 27.13,30.48 29.67,27.94 30.48,27.94 IC1.23
GPA3  (via drill 0.41)
  Top 0.203: v23.37,31.19 19.71,27.53 v16.87,27.53
  Bottom 0.203: v23.37,31.19 27.03,31.19 29.67,28.55 30.48,28.55 IC1.24 | v16.87,27.53 12.19,22.86 B5.P$5
GPA4  (via drill 0.41)
  Top 0.203: v31.9,29.26 30.58,29.26 25.81,34.04 17.48,34.04 11.38,27.94 7.11,27.94 6.4,27.23 6.4,14.43 12.09,8.74 12.09,5.08 B1.P$5
  Bottom 0.203: v31.9,29.26 30.58,29.26 IC1.25
GPA5  (via drill 0.41)
  Top 0.203: v26.72,32.11 20.73,32.11 v17.58,28.96
  Bottom 0.203: v26.72,32.11 28.96,29.87 30.48,29.87 IC1.26 | v17.58,28.96 17.58,18.19 20.83,14.94 20.83,12.7 B2.P$5
GPA6  (via drill 0.41)
  Top 0.203: v48.26,16.97 48.26,13.92 48.97,13.21 48.97,6.3 47.75,5.08 B3.P$5
  Bottom 0.203: v48.26,16.97 48.26,20.52 48.97,21.23 48.97,30.99 48.26,31.7 29.67,31.7 29.46,31.5 29.46,30.79 29.67,30.58 30.48,30.58 IC1.27
GPA7  (via drill 0.41)
  Top 0.203: v36.07,25.6 38.71,25.6 46.63,17.68 48.56,17.68 56.49,9.75 56.49,5.08 B4ALT.P$5 B4.P$5
  Bottom 0.203: v36.07,25.6 36.07,26.82 31.8,31.09 30.58,31.09 IC1.28
GPA12  (via drill 0.41)
  Top 0.203: v41.86,28.45 42.16,28.45 42.67,27.94 72.03,27.94 74.27,25.7 v74.27,25.6
  Bottom 0.203: v41.86,28.45 37.8,28.45 IC1.5 | v74.27,25.6 74.57,25.6 78.54,21.64 84.33,21.64 B9ALT.P$5 84.43,21.64 85.14,22.35 92.25,22.35 92.96,21.64 94.49,21.64 B9.P$5
GPAS0  (via drill 0.41)
  Top 0.203: v93.98,24.28 93.98,23.98 95,22.96 98.55,22.96 101.91,19.61 v101.91,19.2 | v104.34,20.32 104.34,20.73 102.72,22.35 102.72,22.96 105.36,25.6 112.88,25.6 114,26.72 B10.2 | JP3.2 118.67,30.48 117.35,29.16 116.03,29.16 v115.93,29.26
  Bottom 0.203: v93.98,24.28 93.17,25.09 93.17,25.81 IC5.21 | v101.91,19.2 103.33,19.2 104.34,20.22 v104.34,20.32 | v115.93,29.26 115.93,28.65 114.1,26.82 B10.2
GPAS1  (via drill 0.41)
  Top 0.203: v94.49,27.33 99.67,27.33 100.08,27.74 110.44,27.74 v110.74,27.43 | v122.63,21.23 117.65,16.26 116.43,16.26 114.5,14.33 114.1,14.33 B11.2
  Bottom 0.203: v94.49,27.33 93.27,27.33 92.56,26.62 92.56,25.91 IC5.22 | v110.74,27.43 111.15,27.43 115.52,31.8 123.14,31.8 JP3.4 124.36,30.48 122.63,28.75 v122.63,21.23
GPAS2  (via drill 0.41)
  Top 0.203: v91.44,24.49 91.64,24.49 92.35,25.2 96.93,25.2 110.03,12.09 110.03,5.79 113.03,2.79 | 113.03,2.79 114,1.83 B12.2 | JP4.2 118.67,5.08 116.43,2.85 113.08,2.85 113.03,2.79
  Bottom 0.203: v91.44,24.49 91.85,24.89 91.85,25.81 IC5.23
GPAS3  (via drill 0.41)
  Top 0.203: v92.56,27.94 94.08,27.94 94.28,28.14 125.17,28.14 125.63,27.69 | 125.63,27.69 126.49,26.82 B13.2 | JP3.5 127,29.06 125.63,27.69
  Bottom 0.203: v92.56,27.94 91.24,26.62 91.24,25.91 IC5.24
GPAS4  (via drill 0.41)
  Top 0.203: v87.78,31.6 88.19,31.6 89,32.41 97.03,32.41 v99.16,30.28 | v110.13,33.73 110.44,33.73 111.86,35.15 130.66,35.15 132.08,33.73 JP3.7 130.25,28.65 v130.25,28.45
  Bottom 0.203: v87.78,31.6 87.78,25.2 88.29,24.69 90.22,24.69 90.53,24.99 90.53,25.81 IC5.25 | v99.16,30.28 99.16,29.06 100.08,28.14 104.55,28.14 v110.13,33.73 | v130.25,28.45 124.66,28.45 123.34,27.13 123.34,20.93 126.49,17.78 126.49,14.33 B14.2
GPAS5  (via drill 0.41)
  Top 0.203: v90.53,27.23 93.57,27.23 94.79,26.01 96.72,26.01 110.44,12.29 110.44,8.23 111.96,6.71 v115.21,6.71
  Bottom 0.203: v90.53,27.23 89.92,26.62 89.92,25.91 IC5.26 | v115.21,6.71 122.33,6.71 122.63,6.4 125.68,6.4 JP4.5 126.59,5.38 126.59,1.83 B15.2
GPAS6  (via drill 0.41)
  Top 0.203: v90.83,28.55 92.15,28.55 92.25,28.65 99.57,28.65 99.67,28.55 125.48,28.55 v126.09,29.16
  Bottom 0.203: v90.83,28.55 89.31,27.03 89.31,25.91 IC5.27 | v126.09,29.16 133.3,29.16 JP3.8 134.62,30.38 134.93,30.38 138.48,26.82 138.99,26.82 B16.2
GPAS7  (via drill 0.41)
  Top 0.203: v88.7,30.48 89.1,30.48 90.22,31.6 95.81,31.6 v97.43,29.97 | v100.38,27.03 104.85,27.03 105.05,27.23 106.07,27.23 v106.27,27.03 | JP3.10 140.82,30.48 144.07,27.23 144.07,20.83 139.09,15.85 139.09,14.33 B17.2
  Bottom 0.203: v88.7,30.48 88.7,25.91 IC5.28 | v100.38,27.03 v97.43,29.97 | v106.27,27.03 106.27,27.64 110.85,32.21 110.85,34.14 111.86,35.15 134.11,35.15 137.47,31.8 138.38,31.8 JP3.10
GPBS0  (via drill 0.61)
  Top 0.406: v90.73,29.57 91.03,29.57 91.44,29.16 99.77,29.16 v99.97,29.36 | v106.17,30.89 107.59,30.89 v109.12,29.36 | v108.71,23.57 105.36,20.22 105.36,18.19 113.59,9.96 131.06,9.96 131.88,9.14 131.88,7.72 134.52,5.08 JP4.8
  Bottom 0.406: v90.73,29.57 88.59,31.7 88.59,33.02 IC5.1 | v99.97,29.36 100.28,29.36 100.99,28.65 103.94,28.65 v106.17,30.89 | v109.12,29.36 109.12,23.98 v108.71,23.57 | JP4.8 136.04,3.66 136.85,3.66 138.68,1.83 138.99,1.83 B18.2
I2C_SCL  (via drill 0.41)
  Top 0.203: v30.18,17.17 30.18,13.82 | 30.18,13.82 v30.18,11.68 | v87.07,8.64 87.07,9.96 86.92,10.11 | 86.92,10.11 84.73,12.29 83.11,12.29 v81.38,14.02 | v102.11,17.98 102.11,17.68 102.31,17.48 102.31,16.76 95.81,10.26 v93.98,10.26 | 86.92,10.11 v87.17,10.36 | v97.74,34.24 87.68,34.24 84.43,30.99 84.43,23.27 85.65,22.05 85.65,21.13 84.02,19.51 v83.62,19.51 | 30.18,13.82 32.92,13.82 34.24,12.5 34.24,11.18 34.65,10.77 35.97,10.77 41.96,16.76 v41.96,16.97 | v62.08,18.69 v46.63,18.69
  Bottom 0.203: v30.18,11.68 31.19,11.68 IC2.26 | v30.18,17.17 36.98,23.98 37.69,23.98 IC1.12 | v87.07,8.64 91.24,4.47 91.24,2.44 IC3.26 | 78.13,14.02 73.36,14.02 SERIAL.4 73.25,14.12 72.03,15.34 72.03,19.61 71.22,20.42 70.31,20.42 68.58,18.69 v62.08,18.69 | 78.13,14.02 v81.38,14.02 | v102.11,17.98 102.31,17.78 102.31,15.65 IC4.26 | v93.98,10.26 93.67,10.26 93.57,10.36 v87.17,10.36 | v97.74,34.24 96.11,34.24 95.81,33.93 95.81,33.12 IC5.12 | 78.13,14.02 v83.62,19.51 | v41.96,16.97 44.91,16.97 v46.63,18.69
I2C_SDA  (via drill 0.41)
  Top 0.203: v82.19,5.18 81.18,5.18 78.13,8.23 76.1,8.23 v75.08,9.25 75.18,9.25 79.86,13.92 v79.86,14.73 | v101.19,17.68 99.97,18.9 v99.97,19 | v96.72,31.7 96.32,31.7 96.01,32 89.2,32 87.78,30.58 87.78,21.34 v87.68,21.23 | v41.05,16.87 v38.81,19.1
  Bottom 0.203: 37.95,19.96 38.91,20.93 38.91,22.96 38.61,23.27 37.8,23.27 IC1.13 | 37.95,19.96 35.76,17.78 35.76,15.04 32.92,12.19 32.31,12.19 32.21,12.29 31.29,12.29 IC2.27 | v82.19,5.18 83.41,5.18 85.04,3.56 90.02,3.56 90.63,2.95 90.63,2.44 IC3.27 | v75.08,9.25 74.17,10.16 72.85,10.16 72.03,10.97 72.03,12.8 70.81,14.02 SERIAL.3 70.71,14.12 68.58,16.26 41.66,16.26 v41.05,16.87 | v101.19,17.68 101.5,17.37 101.5,15.65 IC4.27 | v99.97,19 98.04,19 96.93,17.88 95,17.88 94.79,18.09 90.32,18.09 89.41,19 87.68,19 | 87.68,19 84.12,19 v79.86,14.73 | v96.72,31.7 96.42,32 96.42,33.02 IC5.13 | 87.68,19 v87.68,21.23 | v38.81,19.1 37.95,19.96
L0
  Bottom 0.203: R20.1 9.25,10.97 8.03,10.97 7.62,11.38 B1.P$2
L1
  Bottom 0.203: R19.1 9.25,6.81 8.03,6.81 7.62,6.4 B1.P$3
L2
  Bottom 0.203: R18.1 23.57,6.81 24.99,6.81 25.4,6.4 B2.P$2
L3
  Bottom 0.203: R17.1 23.57,10.97 24.99,10.97 25.4,11.38 B2.P$3
L4
  Bottom 0.203: R16.1 44.81,10.97 43.59,10.97 43.18,11.38 B3.P$2
L5
  Bottom 0.203: R15.1 44.81,6.81 43.59,6.81 43.18,6.4 B3.P$3
L6
  Bottom 0.203: B4ALT.P$2 52.53,10.97 53.75,10.97 R14.1 53.85,10.87 54.66,10.06 59.64,10.06 60.96,11.38 B4.P$2
L7
  Bottom 0.203: B4ALT.P$3 52.53,6.81 53.75,6.81 R13.1 53.85,6.91 54.66,7.72 59.64,7.72 60.96,6.4 B4.P$3
L8
  Bottom 0.203: R12.1 9.25,28.75 8.03,28.75 7.62,29.16 B5.P$2
L9
  Bottom 0.203: R11.1 9.25,24.59 8.03,24.59 7.62,24.18 B5.P$3
L10
  Bottom 0.203: R10.1 23.57,24.59 24.99,24.59 25.4,24.18 B6.P$2
L11
  Bottom 0.203: R9.1 23.57,28.75 24.99,28.75 25.4,29.16 B6.P$3
L12
  Bottom 0.203: R8.1 44.81,28.75 43.59,28.75 43.18,29.16 B7.P$2
L13
  Bottom 0.203: R7.1 44.81,24.59 43.59,24.59 43.18,24.18 B7.P$3
L14
  Top 0.203: B8ALT.P$2 52.12,29.26 60.96,29.26 B8.P$2
  Bottom 0.203: B8ALT.P$2 52.53,28.75 53.75,28.75 R6.1
L15
  Top 0.203: B8ALT.P$3 52.12,24.18 60.96,24.18 B8.P$3
  Bottom 0.203: B8ALT.P$3 52.53,24.59 53.75,24.59 R5.1
L16  (via drill 0.41)
  Top 0.203: v95.4,15.24 B9.P$2
  Bottom 0.203: B9ALT.P$2 90.93,17.27 R32.1 92.56,17.27 94.59,15.24 v95.4,15.24
L17
  Bottom 0.203: B9ALT.P$3 90.22,19 92.35,19 R31.1 92.46,19 93.78,20.32 B9.P$3
LS0  (via drill 0.41)
  Top 0.203: B10.L2 116.03,26.82 117.96,26.82 B10.L1 118.72,26.06 | v116.53,18.29 119.08,20.83 119.08,25.7 118.72,26.06 | 118.72,26.06 v119.99,27.33
  Bottom 0.203: v116.53,18.29 R34.1 | JP3.3 121.92,29.26 v119.99,27.33
LS1  (via drill 0.41)
  Top 0.203: B11.L1 117.96,14.33 116.03,14.33 B11.L2 | JP4.4 123.75,5.08 122.43,3.76 v118.36,3.76
  Bottom 0.203: B11.L2 115.93,14.22 110.34,8.64 R33.1 110.54,8.74 115.52,3.76 v118.36,3.76
LS2
  Top 0.203: B12.L1 117.96,1.83 116.03,1.83 B12.L2
  Bottom 0.203: R30.1 110.13,7.21 110.54,7.21 115.93,1.83 B12.L2 | JP4.3 121.31,5.08 118.06,1.83 B12.L1
LS3  (via drill 0.41)
  Top 0.203: 129.54,26.82 128.52,26.82 B13.L2 128.42,26.72 127.41,25.7 126.09,25.7 v117.45,17.07 | 129.54,26.82 130.45,26.82 B13.L1 | 129.54,26.82 JP3.6
  Bottom 0.203: v117.45,17.07 112.67,17.07 R29.1
LS4  (via drill 0.41)
  Top 0.203: v111.25,10.57 111.25,9.55 110.85,9.14 110.85,8.43 111.66,7.62 v115.21,7.62 | B14.L1 130.45,14.33 128.52,14.33 B14.L2
  Bottom 0.203: v111.25,10.57 110.74,10.06 110.13,10.06 R28.1 | v115.21,7.62 121.82,7.62 121.87,7.67 | 121.87,7.67 128.42,14.22 B14.L2 | JP4.7 131.37,5.08 128.83,7.62 121.92,7.62 121.87,7.67
LS5
  Top 0.203: 129.54,1.83 128.52,1.83 B15.L2 | 129.54,1.83 130.45,1.83 B15.L1 | 129.54,1.83 JP4.6
  Bottom 0.203: R27.1 110.13,5.79 110.64,5.28 110.74,5.28 110.95,5.08 110.95,2.23 110.85,2.13 110.85,1.42 111.56,0.71 127.41,0.71 128.42,1.73 B15.L2
LS6  (via drill 0.41)
  Top 0.203: B16.L1 142.95,26.82 141.02,26.82 B16.L2 140.92,26.82 140.72,26.82 138.33,29.21 | 138.33,29.21 137.16,30.38 JP3.9 | v118.16,15.75 123.34,20.93 123.34,21.64 127,25.3 130.56,25.3 132.18,26.92 132.18,27.23 134.11,29.16 138.28,29.16 138.33,29.21
  Bottom 0.203: v118.16,15.75 R26.1
LS7  (via drill 0.41)
  Top 0.203: v112.67,11.99 118.36,11.99 119.69,10.67 130.86,10.67 132.89,12.7 139.4,12.7 140.92,14.22 B17.L2 141.02,14.33 142.95,14.33 B17.L1
  Bottom 0.203: v112.67,11.99 112.17,11.48 110.13,11.48 R25.1 | JP4.10 140.82,5.08 144.07,8.33 144.07,13.21 143.05,14.22 B17.L1
LS8  (via drill 0.41)
  Top 0.203: B18.L1 142.95,1.83 141.02,1.83 B18.L2 140.92,1.83 140.51,1.83 137.36,4.98 137.16,4.98 JP4.9 132.79,0.71 111.56,0.71 v110.13,2.13
  Bottom 0.203: v110.13,2.13 110.13,4.37 R24.1
N$1  (via drill 0.41)
  Top 0.203: v108.31,20.12 108.31,18.09 108.92,17.48 108.92,15.75 v110.03,14.63
  Bottom 0.203: v108.31,20.12 108.71,20.52 108.71,21.44 IC4.13 | v110.03,14.63 110.03,13.11 108.41,11.48 R25.2
N$2  (via drill 0.41)
  Top 0.203: v108.81,22.55 108.81,20.62 109.63,19.81 v109.63,16.76
  Bottom 0.203: v108.81,22.55 108.71,22.55 108.1,21.95 108.1,21.54 IC4.12 | v109.63,16.76 110.64,15.75 R26.2
N$3  (via drill 0.41)
  Top 0.203: v95.5,30.89 90.12,30.89 89,29.77 v89,23.98 | v90.53,23.37 90.53,22.05 92.96,19.61 v96.22,19.61 | v97.64,19.61 97.64,17.48 98.65,16.46 v99.97,16.46 | v101.09,10.67 102.72,10.67 107.09,6.3 v107.19,6.3
  Bottom 0.203: v95.5,30.89 100.79,25.6 106.68,25.6 107.8,24.49 107.8,23.47 107.49,23.16 107.49,21.54 IC4.11 | v89,23.98 89.92,23.98 v90.53,23.37 | v97.64,19.61 v96.22,19.61 | v99.97,16.46 99.97,16.05 100.28,15.75 100.28,11.48 v101.09,10.67 | v107.19,6.3 107.9,6.3 108.31,5.89 R27.2
N$4
  Bottom 0.203: IC2.13 37.08,5.08 42.06,5.08 43.28,3.86 52.53,3.86 55.47,6.81 R13.2
N$5  (via drill 0.41)
  Top 0.203: v35.97,5.89 35.97,6.91 42.06,13.01 v42.06,13.82 | v56.59,10.97 v53.65,13.92
  Bottom 0.203: v35.97,5.89 36.98,5.89 IC2.12 | v42.06,13.82 47.04,13.82 47.14,13.92 v53.65,13.92 | v56.59,10.97 55.58,10.97 R14.2
N$6  (via drill 0.41)
  Top 0.203: v103.73,17.37 103.73,14.53 107.19,11.07 v107.19,10.77
  Bottom 0.203: v103.73,17.37 103.94,17.58 105.66,17.58 106.88,18.8 106.88,19.41 106.78,19.51 106.78,21.44 IC4.10 | v107.19,10.77 107.49,10.77 108.31,9.96 R28.2
N$7
  Bottom 0.203: IC2.11 37.08,6.4 41.35,6.4 42.67,5.08 44.81,5.08 46.53,6.81 R15.2
N$8  (via drill 0.41)
  Top 0.203: v107.9,17.48 v106.17,19.2
  Bottom 0.203: v106.17,19.2 106.17,21.44 IC4.9 | v107.9,17.48 110.44,17.48 110.85,17.07 R29.2
N$9  (via drill 0.41)
  Top 0.203: v39.73,7.21 42.67,10.16 43.69,10.16 v45.52,11.99
  Bottom 0.203: v39.73,7.21 37.08,7.21 IC2.10 | v45.52,11.99 46.53,10.97 R16.2
N$10  (via drill 0.41)
  Top 0.203: v35.76,7.72 30.68,7.72 29.97,7.01 27.84,7.01 25.91,5.08 24.89,5.08 22.45,7.52 v22.45,9.86
  Bottom 0.203: v35.76,7.72 36.98,7.72 IC2.9 | v22.45,9.86 22.45,10.26 21.84,10.87 R17.2
N$11  (via drill 0.41)
  Top 0.203: v34.24,8.43 30.79,8.43 29.97,7.62 23.47,7.62 v23.16,7.92
  Bottom 0.203: v34.24,8.43 36.98,8.43 IC2.8 | v23.16,7.92 22.86,7.92 21.84,6.91 R18.2
N$12  (via drill 0.41)
  Top 0.203: v38.71,7.92 38.71,7.01 33.22,1.52 17.48,1.52 v13.61,5.38
  Bottom 0.203: v38.71,7.92 37.59,9.04 37.08,9.04 IC2.7 | v13.61,5.38 12.19,6.81 11.07,6.81 R19.2
N$13  (via drill 0.41)
  Top 0.203: v94.59,29.97 91.44,29.97 90.93,30.48 90.32,30.48 89.71,29.87 89.71,21.23 90.12,20.83 v90.12,13.01 | v91.44,11.68 91.44,10.46 92.96,8.94 95.5,8.94 98.04,11.48 102.92,11.48 v107.19,7.21
  Bottom 0.203: v94.59,29.97 95.81,29.97 100.58,25.2 106.48,25.2 107.39,24.28 107.39,23.67 106.98,23.27 106.78,23.27 105.56,22.05 105.56,21.54 IC4.8 | v91.44,11.68 v90.12,13.01 | v107.19,7.21 108.31,7.21 R30.2
N$14  (via drill 0.41)
  Top 0.203: v95.3,18.59 v91.75,15.04
  Bottom 0.203: v91.75,15.04 93.78,13.01 93.78,11.48 94.69,10.57 94.69,9.96 93.98,9.25 93.98,8.33 IC3.7 | v95.3,18.59 94.49,18.59 94.18,18.9 R31.2
N$15  (via drill 0.41)
  Top 0.203: v93.27,9.65 93.27,10.57 93.78,11.07 93.78,13.01 93.27,13.51 93.27,14.53 v94.79,16.05
  Bottom 0.203: v93.27,9.65 93.27,8.33 IC3.6 | v94.79,16.05 94.79,16.66 94.18,17.27 R32.2
N$16  (via drill 0.41)
  Top 0.203: v103.02,17.98 103.02,12.39 v107.19,8.23
  Bottom 0.203: v103.02,17.98 105.05,20.02 105.05,20.62 104.85,20.83 104.85,21.44 IC4.7 | v107.19,8.23 107.9,8.23 108.31,8.64 R33.2
N$17  (via drill 0.41)
  Top 0.203: v106.68,23.98 107.8,25.09 v113.79,25.09 | v111.96,23.27 111.96,22.76 110.85,21.64 v110.85,19.41
  Bottom 0.203: v106.68,23.98 105.77,23.06 105.26,23.06 104.24,22.05 104.24,21.54 IC4.6 | v111.96,23.27 v113.79,25.09 | v110.85,19.41 110.85,18.29 R34.2
N$18
  Bottom 0.203: IC4.15 109.32,15.54 109.32,13.92 106.48,11.07 106.48,5.99 108,4.47 108.31,4.47 R24.2
N$19  (via drill 0.41)
  Top 0.203: v34.14,9.55 31.29,9.55 30.07,8.33 27.74,8.33 25.91,10.16 23.16,10.16 22.35,10.97 v15.04,10.97
  Bottom 0.203: v34.14,9.55 34.24,9.65 36.98,9.65 IC2.6 | v15.04,10.97 11.07,10.97 R20.2
N$20  (via drill 0.41)
  Top 0.203: v25.6,3.56 19.51,3.56 10.87,12.19 v10.87,25.91
  Bottom 0.203: v25.6,3.56 26.52,4.47 31.19,4.47 IC2.15 | v10.87,25.91 10.87,28.55 10.97,28.65 R12.2
N$21  (via drill 0.41)
  Top 0.203: v22.45,5.18 22.45,6.3 v18.49,10.26
  Bottom 0.203: v22.45,5.18 22.96,4.67 26.11,4.67 26.52,5.08 31.19,5.08 IC2.16 | v18.49,10.26 18.49,11.68 15.04,15.14 15.04,17.78 10.87,21.95 10.87,24.49 10.97,24.59 R11.2
N$22  (via drill 0.41)
  Top 0.203: v23.16,5.79 23.16,6.2 21.34,8.03 v21.34,9.86 | v17.98,13.21 17.98,21.74 v20.62,24.38
  Bottom 0.203: v23.16,5.79 23.88,5.08 25.91,5.08 26.62,5.79 31.19,5.79 IC2.17 | v17.98,13.21 v21.34,9.86 | v20.62,24.38 21.54,24.38 21.74,24.59 R10.2
N$23
  Bottom 0.203: IC2.18 31.29,6.4 31.8,6.4 32.11,6.1 32.11,4.27 31.29,3.45 26.52,3.45 24.59,1.52 10.67,1.52 6.4,5.79 6.4,29.77 8.33,31.7 17.88,31.7 20.83,28.75 21.74,28.75 R9.2
N$24  (via drill 0.41)
  Top 0.203: v28.35,13.31 v28.35,9.45 | v40.44,21.64 v36.68,21.64
  Bottom 0.203: v28.35,9.45 30.58,7.21 31.19,7.21 IC2.19 | v36.68,21.64 v28.35,13.31 | v40.44,21.64 40.44,23.16 42.67,25.4 43.69,25.4 46.53,28.25 46.53,28.65 R8.2
N$25  (via drill 0.41)
  Top 0.203: v32.92,5.28 33.63,4.57 35.66,4.57 38,6.91 38,8.33 42.77,13.11 v42.77,20.42
  Bottom 0.203: v32.92,5.28 32.92,6.6 31.8,7.72 31.29,7.72 IC2.20 | v42.77,20.42 46.53,24.18 46.53,24.59 R7.2
N$26  (via drill 0.41)
  Top 0.203: v29.77,9.04 29.77,11.07 29.46,11.38 29.46,22.96 31.6,25.09 35.56,25.09 38.3,22.35 40.95,22.35 v41.35,21.95 | v44.91,23.57 46.63,23.57 47.45,24.38 v50.6,24.38
  Bottom 0.203: v29.77,9.04 30.38,8.43 31.19,8.43 IC2.21 | v41.35,21.95 43.28,21.95 v44.91,23.57 | v50.6,24.38 51.61,25.4 52.53,25.4 55.47,28.35 55.47,28.65 R6.2
N$27  (via drill 0.41)
  Top 0.203: v28.96,27.64 33.22,27.64 34.34,28.75 40.13,28.75 41.96,26.92 41.96,26.11 42.67,25.4 54.15,25.4 v54.46,25.7 | v29.06,26.01 v29.06,10.77
  Bottom 0.203: v29.06,10.77 30.68,9.14 31.19,9.14 IC2.22 | v29.06,26.01 29.06,27.53 v28.96,27.64 | v54.46,25.7 55.47,24.69 R5.2
SLIDER_IN
  Top 0.203: 76.81,22.25 74.68,22.25 72.03,19.61 72.03,18.59 70.81,17.37 70.81,16.66 SERIAL.5 | 76.81,22.25 80.57,26.01 JP1.2 | 80.57,15.85 80.57,18.49 76.81,22.25 | 80.57,15.85 80.57,9.55 JP2.2 | 80.57,15.85 83.72,12.7 85.85,12.7 87.88,10.67 87.88,4.67 84.63,1.42 83.72,1.42 POT1.2A
  Bottom 0.203: C6.1 81.18,3.66 81.38,3.66 83.62,1.42 POT1.2A

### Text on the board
_bsilk: v08-13 | PCB-CMB-3 | SKAARHOJ 2013 | GITHUB: SKAARHOJ-Open-Engineering

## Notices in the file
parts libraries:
SparkFun: Licensing: CC v3.0 Share-Alike You are welcome to use this library for commercial purposes.
